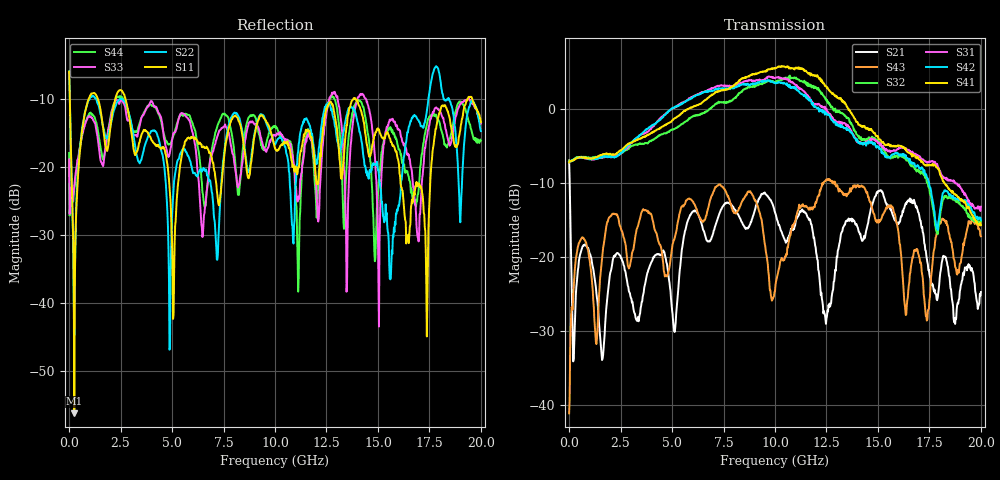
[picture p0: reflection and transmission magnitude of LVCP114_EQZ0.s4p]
!Agilent Technologies,N5230A,MY46400459,A.07.50.48
!Agilent N5230A: A.07.50.48
!Date: Monday, January 09, 2012 14:01:10
!Correction: S11(Full 4 Port(1,2,3,4))
!S12(Full 4 Port(1,2,3,4))
!S13(Full 4 Port(1,2,3,4))
!S14(Full 4 Port(1,2,3,4))
!S21(Full 4 Port(1,2,3,4))
!S22(Full 4 Port(1,2,3,4))
!S23(Full 4 Port(1,2,3,4))
!S24(Full 4 Port(1,2,3,4))
!S31(Full 4 Port(1,2,3,4))
!S32(Full 4 Port(1,2,3,4))
!S33(Full 4 Port(1,2,3,4))
!S34(Full 4 Port(1,2,3,4))
!S41(Full 4 Port(1,2,3,4))
!S42(Full 4 Port(1,2,3,4))
!S43(Full 4 Port(1,2,3,4))
!S44(Full 4 Port(1,2,3,4))
!S4P File: Measurements: <S11,S12,S13,S14>,
!<S21,S22,S23,S24>,
!<S31,S32,S33,S34>,
!<S41,S42,S43,S44>:
# Hz S  dB  R 50
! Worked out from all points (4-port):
!   801 points, 300 kHz to 20 GHz, reference 50 ohm
!   strongest paths, dB at 300 kHz, 5 GHz, 10 GHz, 15 GHz, 20 GHz:
!     S41: -7.3, -1.6, 5.5, -3.7, -15.7
!     S42: -7.1, 0.0, 3.5, -5.1, -15.0
!     S31: -7.2, 0.0, 4.1, -4.7, -13.3
!     S32: -7.0, -2.8, 3.5, -4.6, -15.2
!     S43: -41.2, -18.9, -24.7, -15.2, -17.2
!     S21: -7.0, -27.2, -14.0, -11.2, -24.8
!   lowest |S11| = -56.2 dB at 250.3 MHz (marker M1), VSWR 1.00, Z = 50.2 - j0.0295 ohm
!   |S11| at or under -10 dB: 34.69 MHz to 946.3 MHz (911.6 MHz wide, 186 % of centre); 2.738 GHz to 13.81 GHz (11.07 GHz wide, 134 % of centre); 13.92 GHz to 19.36 GHz (5.441 GHz wide, 32.7 % of centre)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
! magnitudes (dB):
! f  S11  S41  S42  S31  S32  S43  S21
! 300 kHz  -6.0  -7.3  -7.1  -7.2  -7.0  -41.2  -7.0
! 250.3 MHz  -56.2  -6.9  -6.8  -7.0  -6.8  -22.8  -31.5
! 1.15 GHz  -9.1  -6.7  -6.8  -6.9  -6.6  -24.6  -21.4
! 4.9 GHz  -23.9  -1.8  -0.2  -0.2  -3.0  -20.9  -24.2
! 13.9 GHz  -9.9  -1.5  -4.0  -3.9  -3.1  -10.4  -15.6
! 17.38 GHz  -44.9  -7.7  -9.2  -7.3  -10.0  -28.6  -20.3
! 20 GHz  -13.4  -15.7  -15.0  -13.3  -15.2  -17.2  -24.8
